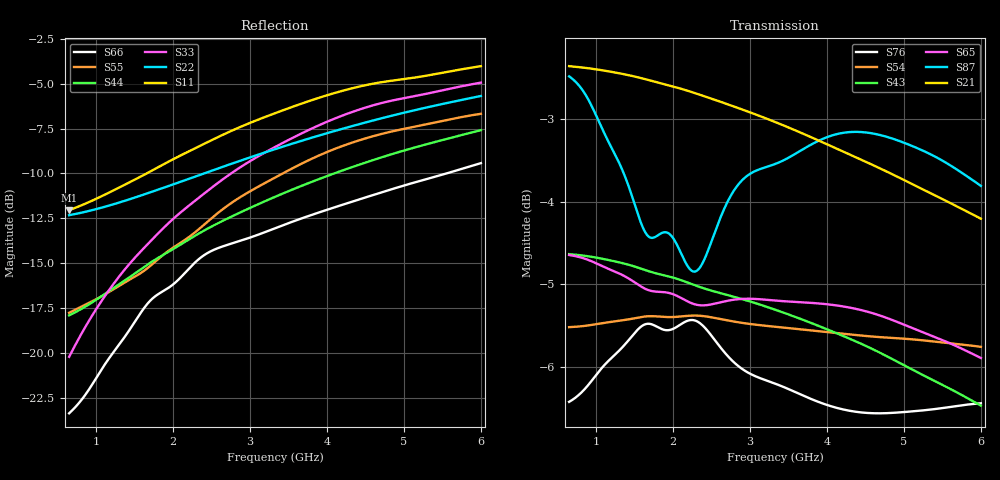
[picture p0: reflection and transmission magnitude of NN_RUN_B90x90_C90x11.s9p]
! IGNION VIRTUAL ANTENNA LIBRARY
! NN_RUN_B90x90_C90x11
! Virtual Antenna™ RUN mXTEND™: NN02-224 12.0 mm x 3.0 mm x 2.4 mm
! https://ignion.io/product/run-mxtend/
! Board: 90 mm x 90 mm
! Clearance Area: 90 mm x 11 mm
! Feeding line: L-shape; 11mm x 2mm and 5mm x 2mm
! Applications: Fleet management, IoT
! Frequency range 0.65GHz to 6GHz, step 10MHz
! Number of ports 9
! This product and its use is protected by at least one or more of the following patents and patent
! applications US 8,203,492 B2; US 8,237,615 B2; PCT/EP2013/064692; WO 2014/012842 A1; US 2019/190122 A1;
! US 62/072,671; and other domestic and international patents pending. Additional information about
! patents related to this product is available at https://ignion.io/files/Patent-list-NN.pdf, all
! rights reserved. Copyright, Ignion 2021.
! Need more help? Your platform is much different than these examples in the manual? Use our
! Fast Track service (https://ignion.io/fast-track/), for free, and get a personalized antenna design in
! just 24 hours.
! Touchstone port 1 = "Series Port"
! Touchstone port 2 = "Shunt Port"
! Touchstone port 3 = "Series Port"
! Touchstone port 4 = "Shunt Port"
! Touchstone port 5 = "Series Port"
! Touchstone port 6 = "Shunt Port"
! Touchstone port 7 = "Series Port"
! Touchstone port 8 = "Shunt Port"
! Touchstone port 9 = "Series Port"
! IE3D S-Parameters Output Version 2.0
# GHZ S MA R 50
! Nport = 9
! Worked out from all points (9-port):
!   536 points, 650 MHz to 6 GHz, reference 50 ohm
!   strongest paths, dB at 650 MHz, 1.99 GHz, 3.33 GHz, 4.67 GHz, 6 GHz:
!     S21: -2.4, -2.6, -3.0, -3.6, -4.2
!     S87: -2.5, -4.4, -3.5, -3.2, -3.8
!     S65: -4.6, -5.1, -5.2, -5.4, -5.9
!     S43: -4.6, -4.9, -5.3, -5.8, -6.5
!     S54: -5.5, -5.4, -5.5, -5.6, -5.8
!     S76: -6.4, -5.5, -6.2, -6.6, -6.4
!   lowest |S11| = -12.0 dB at 650 MHz (marker M1), VSWR 1.67, Z = 31.1 + j7.72 ohm
!   |S11| at or under -10 dB: start of sweep to 1.658 GHz
